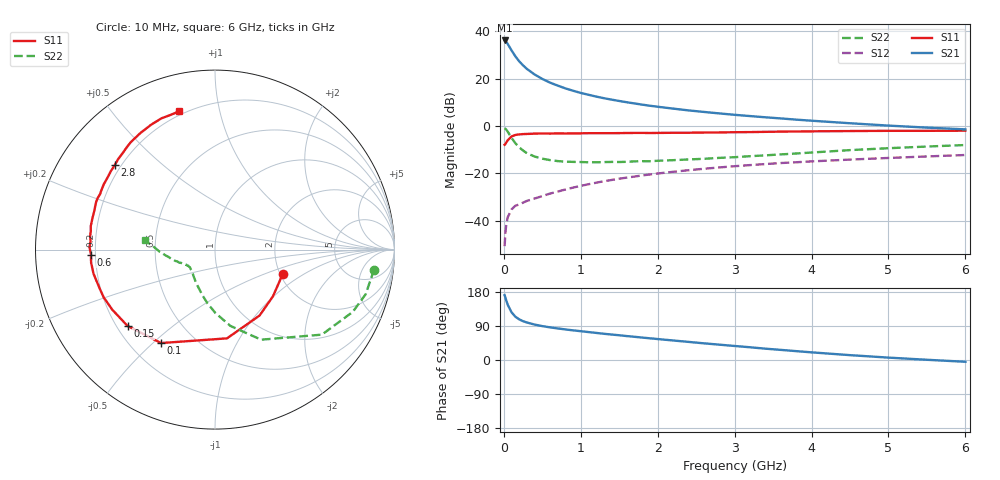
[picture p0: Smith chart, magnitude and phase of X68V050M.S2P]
! SIEMENS Small Signal Semiconductors
! BFP193W
! Si NPN RF Bipolar Junction Transistor in SOT343
! VCE = 8 V  IC = 50 mA
! Common Emitter S-Parameters:  April 1994
# GHz  S  MA  R  50
!  f  S11  S21  S12  S22
! GHz  MAG  ANG  MAG  ANG  MAG  ANG  MAG  ANG
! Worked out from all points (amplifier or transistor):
!   40 points, 10 MHz to 6 GHz, reference 50 ohm
!   highest |S21| = 36.1 dB at 10 MHz (marker M1)
!   |S21| within 3 dB of that: start of sweep to 78.29 MHz
!   unconditionally stable (mu >= 1): 706.1 MHz to 4.504 GHz
!   at 200 MHz: K = 0.53, MSG = 30.2 dB, |S12| = -33.1 dB
!   at 1.5 GHz: K = 1.11, MAG = 14.4 dB, |S12| = -22.3 dB
!   at 6 GHz: K = 0.96, MSG = 5.4 dB, |S12| = -12.3 dB
!   S11 on the Smith chart (normalised r, x): 10 MHz: 2.07, -0.67; 100 MHz: 0.33, -0.53; 150 MHz: 0.24, -0.36; 600 MHz: 0.18, -0.02; 2.8 GHz: 0.18, +0.36; 6 GHz: 0.18, +0.76
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0.01  0.4014 -19.6  63.94 171.1  0.0029 82.2  0.893 -7.2
0.02  0.4148 -38.9  62.46 164.8  0.0055 75.4  0.8756 -16.5
0.03  0.4433 -55.9  60.39 158.0  0.0078 72.5  0.8425 -24.3
0.05  0.499 -82.3  54.12 146.0  0.0118 62.1  0.761 -38.5
0.1  0.6013 -120.0  39.47 125.9  0.0173 49.3  0.5638 -62.9
0.15  0.6468 -138.9  29.56 114.2  0.0207 44.5  0.433 -78.7
0.2  0.6631 -149.7  23.16 107.2  0.0221 44.3  0.3526 -89.7
0.25  0.6749 -156.8  19.04 102.4  0.0241 44.4  0.3035 -97.8
0.3  0.6785 -161.7  16.02 98.9  0.0262 46.3  0.2663 -104.8
0.4  0.69 -168.8  12.22 93.5  0.0294 49.4  0.2261 -115.0
0.5  0.6942 -174.0  9.856 89.4  0.0331 52.3  0.2041 -122.8
0.6  0.6916 -177.7  8.235 86.1  0.0374 54.5  0.1904 -128.8
0.8  0.695 176.2  6.222 80.7  0.0456 58.1  0.1763 -136.4
1.1  0.7043 169.4  4.563 73.7  0.0589 60.1  0.1712 -143.8
1.3  0.7052 165.2  3.864 69.2  0.0681 60.4  0.1728 -146.4
1.6  0.7109 159.6  3.168 63.1  0.0813 59.9  0.1751 -149.4
2.2  0.7189 149.6  2.328 51.5  0.1077 57.1  0.1897 -155.1
2.8  0.7304 139.8  1.843 40.5  0.1332 53.2  0.212 -159.9
3.2  0.7433 134.0  1.62 33.6  0.1494 50.2  0.2301 -164.1
4.5  0.7815 117.1  1.142 12.8  0.1953 40.7  0.3096 -177.9
5.5  0.7901 108.4  0.923 0.6  0.2274 34.1  0.3681 174.7
6  0.7959 104.4  0.848 -4.7  0.2439 31.4  0.3961 172.1
